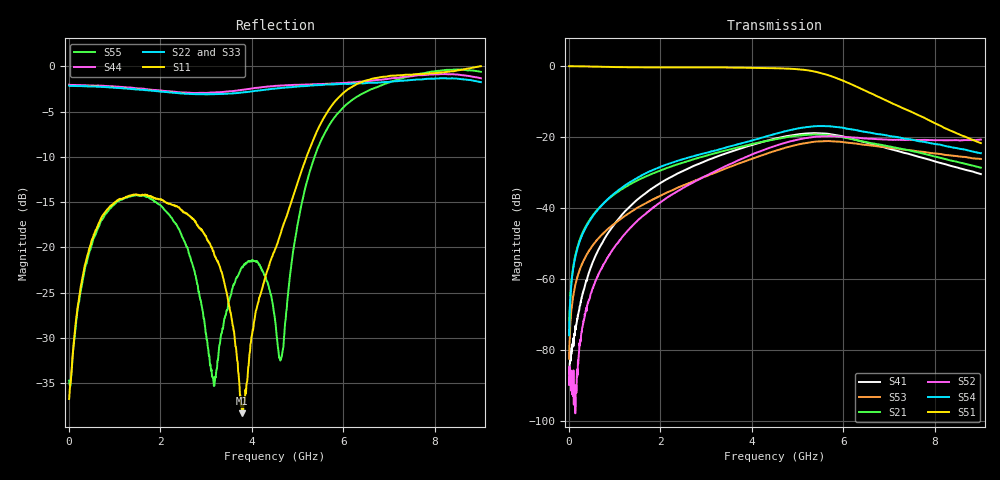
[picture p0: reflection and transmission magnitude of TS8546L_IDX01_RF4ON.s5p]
# GHz S DB R 50
! CMT, SN0916, 25263762, 26.7.0
! Date: 16.07.2026 12:22:20
! Data: Format
! Freq S1.1:dB/Ang S1.2:dB/Ang S1.3:dB/Ang S1.4:dB/Ang S1.5:dB/Ang
!  S2.1:dB/Ang S2.2:dB/Ang S2.3:dB/Ang S2.4:dB/Ang S2.5:dB/Ang
!  S3.1:dB/Ang S3.2:dB/Ang S3.3:dB/Ang S3.4:dB/Ang S3.5:dB/Ang
!  S4.1:dB/Ang S4.2:dB/Ang S4.3:dB/Ang S4.4:dB/Ang S4.5:dB/Ang
!  S5.1:dB/Ang S5.2:dB/Ang S5.3:dB/Ang S5.4:dB/Ang S5.5:dB/Ang
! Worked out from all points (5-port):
!   2001 points, 10 MHz to 9 GHz, reference 50 ohm
!   strongest paths, dB at 10 MHz, 2.257 GHz, 4.505 GHz, 6.753 GHz, 9 GHz:
!     S51: -0.2, -0.5, -0.8, -8.8, -21.8
!     S54: -75.8, -27.3, -19.2, -19.3, -24.6
!     S52: -89.8, -36.3, -22.6, -20.7, -20.8
!     S21: -75.3, -28.3, -20.7, -22.2, -28.7
!     S53: -82.5, -35.1, -24.0, -22.7, -26.3
!     S41: -85.9, -31.2, -20.5, -22.6, -30.5
!   lowest |S11| = -38.3 dB at 3.79 GHz (marker M1), VSWR 1.02, Z = 50.5 - j1.12 ohm
!   |S11| at or under -10 dB: start of sweep to 5.192 GHz
